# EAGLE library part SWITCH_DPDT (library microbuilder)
Switch - DPDT A DPDT Switch acts like an SPDT switch, but has a pair of switches instead of just one. Vertical - 0.3A @ 6V SMT - Digikey: JS202011SCQN
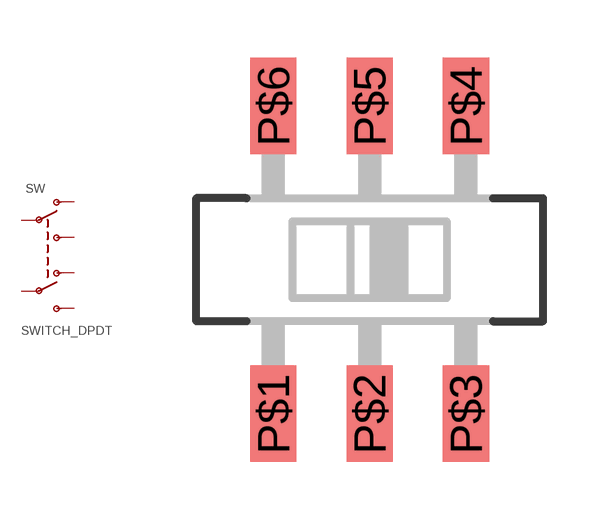
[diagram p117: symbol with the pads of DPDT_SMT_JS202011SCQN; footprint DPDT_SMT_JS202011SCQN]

Designator prefix SW

## SWITCH_DPDT  [DPDT_SMT_JS202011SCQN]
P$1  O1  pas
P$2  P1  pas
P$3  S1  pas
P$4  S2  pas
P$5  P2  pas
P$6  O2  pas

## Footprint DPDT_SMT_JS202011SCQN (pad centres in mm)
smd 1.2 x 2.5: P$1 -2.5,-4; P$2 0,-4; P$3 2.5,-4; P$4 2.5,4; P$5 0,4; P$6 -2.5,4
